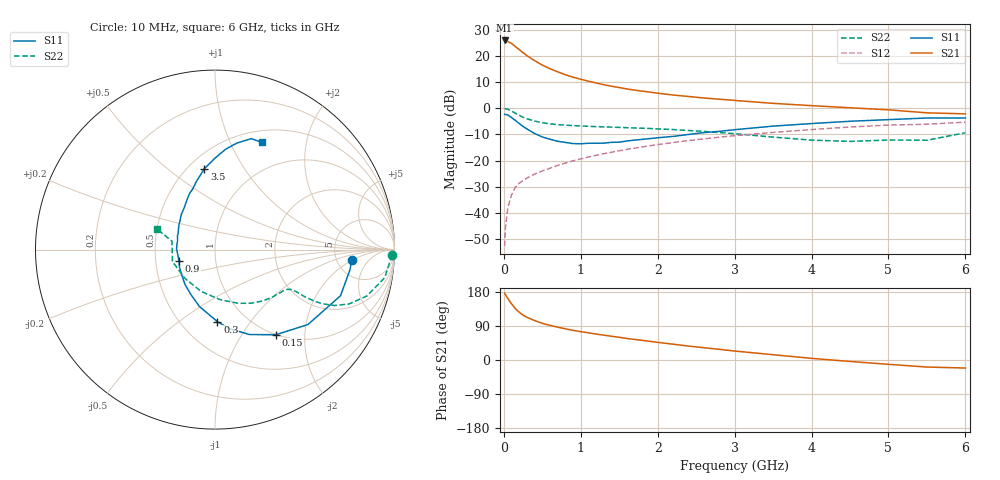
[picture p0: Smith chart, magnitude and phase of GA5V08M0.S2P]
! Infineon Technologies  Discrete & RF Semiconductors
! BF775
! Si NPN RF Bipolar Junction Transistor in SOT23
! VCE = 5 V  IC = 8 mA
! Common Emitter S-Parameters:  May  1996
# GHz  S  MA  R  50
!  f  S11  S21  S12  S22
! GHz  MAG  ANG  MAG  ANG  MAG  ANG  MAG  ANG
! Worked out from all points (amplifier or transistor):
!   36 points, 10 MHz to 6 GHz, reference 50 ohm
!   highest |S21| = 25.9 dB at 10 MHz (marker M1)
!   |S21| within 3 dB of that: start of sweep to 179 MHz
!   unconditionally stable (mu >= 1): 660.9 MHz to 3.054 GHz
!   at 250 MHz: K = 0.61, MSG = 24.4 dB, |S12| = -27.6 dB
!   at 1.4 GHz: K = 1.11, MAG = 10.6 dB, |S12| = -16.8 dB
!   at 6 GHz: K = 0.93, MSG = 1.6 dB, |S12| = -5.3 dB
!   S11 on the Smith chart (normalised r, x): 10 MHz: 6.98, -1.88; 150 MHz: 1.00, -1.44; 300 MHz: 0.74, -0.71; 900 MHz: 0.66, -0.09; 3.5 GHz: 0.60, +0.68; 6 GHz: 0.64, +1.32
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0.01  0.7646 -4.2  19.79 176.3  0.0023 89.8  0.9886 -1.8
0.02  0.7604 -8.5  19.46 172.6  0.005 85.4  0.9773 -3.8
0.05  0.745 -20.2  18.99 163.0  0.0121 79.2  0.9586 -9.4
0.1  0.665 -38.9  17.35 148.2  0.0222 71.8  0.8844 -17.0
0.15  0.5836 -54.3  15.12 135.5  0.0307 66.4  0.8057 -22.1
0.2  0.5115 -67.8  13.26 126.1  0.0366 63.6  0.7343 -25.1
0.25  0.4482 -79.6  11.55 118.4  0.0416 61.3  0.6723 -26.7
0.3  0.4014 -88.1  10.14 112.7  0.0461 61.0  0.6282 -27.4
0.4  0.329 -105.2  8.129 104.1  0.0551 60.9  0.5684 -27.7
0.5  0.282 -119.0  6.679 96.8  0.0631 61.3  0.5281 -27.5
0.6  0.2555 -131.1  5.707 91.4  0.0714 62.3  0.5039 -27.4
0.7  0.2336 -142.2  4.964 86.6  0.0804 62.8  0.4869 -27.5
0.9  0.2109 -162.3  3.931 78.3  0.0988 63.2  0.4654 -28.4
1.1  0.2141 179.2  3.291 71.7  0.1169 63.3  0.4514 -30.2
1.3  0.2146 166.3  2.818 65.5  0.1355 62.5  0.4395 -32.2
1.6  0.2363 149.2  2.336 56.8  0.1633 60.9  0.4241 -36.4
2.2  0.2894 126.4  1.788 41.7  0.2209 56.1  0.3911 -47.0
2.8  0.3612 109.9  1.489 28.2  0.2794 50.0  0.3426 -60.8
3.5  0.455 97.5  1.24 13.9  0.3449 41.8  0.2806 -84.0
4.5  0.5636 83.8  1.021 -3.9  0.437 29.1  0.2321 -136.5
5.5  0.6505 71.9  0.817 -18.6  0.4945 14.2  0.2442 168.9
6  0.6517 66.5  0.781 -21.2  0.5416 10.1  0.3399 160.7
